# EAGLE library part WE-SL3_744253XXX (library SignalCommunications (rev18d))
SMD Common Mode Line Filter WE-SL3 - Small size - Low Profile, only 2.5 mm - High Impedance tp to 5000 ohm - High Current up to 700mA - Low leakage inductance - USB - CAN - Firewire - Data Lines - Power Lines Details see: http://katalog.we-online.de/en/pbs/WE-SL3? Updated by Dan Xu 2014-07-11 2014 (C) Würth Elektronik
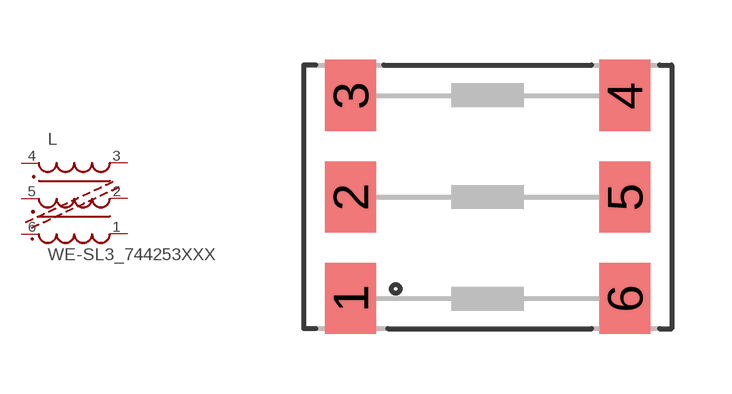
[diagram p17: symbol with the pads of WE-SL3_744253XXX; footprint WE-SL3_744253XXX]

Designator prefix L

## WE-SL3_744253XXX_744253101 (WE-NUMBER: 744253101/100uH), WE-SL3_744253XXX_744253200 (WE-NUMBER: 744253200/20uH)  [WE-SL3_744253XXX]
1  1  pas
2  2  pas
3  3  pas
4  4  pas
5  5  pas
6  6  pas

## Footprint WE-SL3_744253XXX (pad centres in mm)
SMD Common-Mode Line Filter WE-SL3
smd 1.27 x 1.78: 1 -3.43,-2.54; 2 -3.43,0; 3 -3.43,2.54; 4 3.43,2.54; 5 3.43,0; 6 3.43,-2.54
